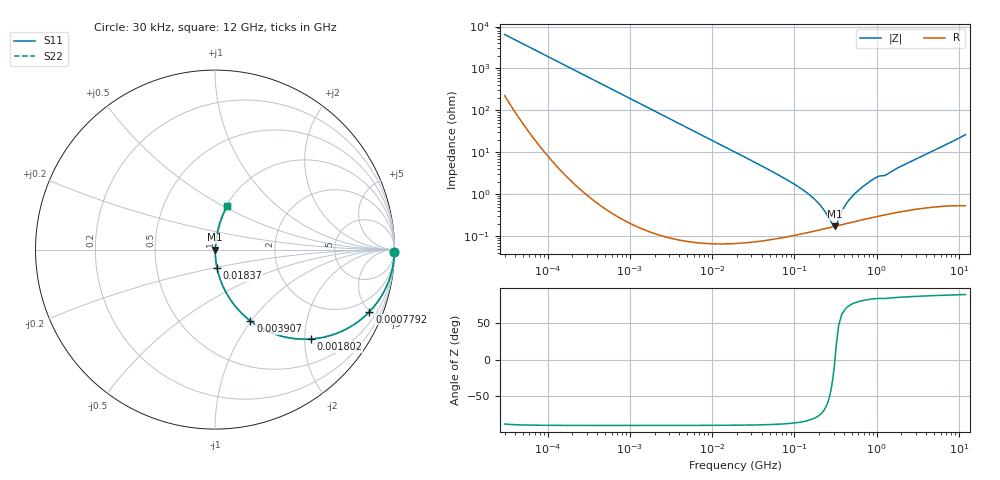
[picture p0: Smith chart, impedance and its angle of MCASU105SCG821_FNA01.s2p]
! MCASU105SCG821_FNA01  S-PARAMETER MODEL  ( General Type )
! Model Generated by TAIYO YUDEN Corporation (http://www.ty-top.com)
! Version 1.0
! TAIYO YUDEN Control No. 130207
! Copyright(c) 2013 TAIYO YUDEN CO.,LTD. All Rights Reserved.
! Product Description (link to TY-COMPAS)
! https://ds.yuden.co.jp/TYCOMPAS/or/detail?pn=MCASU105SCG821JFNA01&u=M
! Products Name : Multilayer Ceramic Capacitors
! Characteristics :
!  Capacitance : 820 pF , Rated Voltage : 50V , TCC : CG / C0G
!  Case Size : 1.0 x 0.5 / 0.039 x 0.02 [mm/inch] , Thickness : 0.5 / 0.02 [mm/inch]
!  (Conditions: Temperature = 25 degC , DC Bias Current/Voltage = 0A / 0V)
! External Node Assignments :
!  1  o---| |---o  2
! GND o---------o GND
! Frequency Range : 30000Hz  -  12GHz  [ 401 STEP ]
# MHz S RI R 50
! Freq[MHz].  S11 Real  S11 Imag  S21 Real  S21 Imag  S12 Real  S12 Imag  S22 Real  S22 Imag
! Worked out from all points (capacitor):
!   401 points, 30 kHz to 12 GHz, reference 50 ohm
!   read as one part in series: C = 821 pF near 32 kHz
!   lowest |Z| = 174 mohm at 313.8 MHz (marker M1)
!   series resonance near 311.2 MHz, so ESL is about 320 pH
!   S11 on the Smith chart (normalised r, x): 30 kHz: open; 779.2 kHz: 1.01, -4.97; 1.802 MHz: 1.00, -2.15; 3.907 MHz: 1.00, -0.99; 18.37 MHz: 1.00, -0.21; 12 GHz: 1.01, +0.53
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0.03  0.9992 -0.0154  0.000776 0.0154  0.000776 0.0154  0.9992 -0.0154
0.260295  0.9821 -0.1319  0.0179 0.1319  0.0179 0.1319  0.9821 -0.1319
0.779186  0.8606 -0.3459  0.1394 0.3459  0.1394 0.3459  0.8606 -0.3459
1.147369  0.7402 -0.438  0.2598 0.438  0.2598 0.438  0.7402 -0.438
1.802085  0.5362 -0.4981  0.4638 0.4981  0.4638 0.4981  0.5362 -0.4981
2.258455  0.4241 -0.4936  0.5759 0.4936  0.5759 0.4936  0.4241 -0.4936
3.907499  0.1977 -0.3975  0.8023 0.3975  0.8023 0.3975  0.1977 -0.3975
7.447352  0.0639 -0.2433  0.9361 0.2433  0.9361 0.2433  0.0639 -0.2433
18.37156  0.0116 -0.1038  0.9884 0.1038  0.9884 0.1038  0.0116 -0.1038
18.97367  0.0109 -0.1006  0.9891 0.1006  0.9891 0.1006  0.0109 -0.1006
80.98098  0.00147 -0.0223  0.9985 0.0223  0.9985 0.0223  0.00147 -0.0223
164.6252  0.00137 -0.0085  0.9986 0.0085  0.9986 0.0085  0.00137 -0.0085
220.0608  0.00149 -0.00445  0.9985 0.00445  0.9985 0.00445  0.00149 -0.00445
294.1636  0.00169 -0.000785  0.9983 0.000785  0.9983 0.000785  0.00169 -0.000785
313.7612  0.00174 0.000133  0.9983 -0.000133  0.9983 -0.000133  0.00174 0.000133
334.6645  0.00179 0.0012  0.9982 -0.0012  0.9982 -0.0012  0.00179 0.0012
406.107  0.00198 0.0047  0.998 -0.0047  0.998 -0.0047  0.00198 0.0047
542.8588  0.00234 0.0101  0.9977 -0.0101  0.9977 -0.0101  0.00234 0.0101
939.2353  0.00342 0.0235  0.9966 -0.0235  0.9966 -0.0235  0.00342 0.0235
1428.372  0.00444 0.0321  0.9956 -0.0321  0.9956 -0.0321  0.00444 0.0321
5023.914  0.0172 0.1098  0.9828 -0.1098  0.9828 -0.1098  0.0172 0.1098
12000  0.0696 0.2445  0.9304 -0.2445  0.9304 -0.2445  0.0696 0.2445
